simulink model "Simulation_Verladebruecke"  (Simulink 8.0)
settings: Solver=ode23  StartTime=0.0  StopTime=20  RelTol=1e-3
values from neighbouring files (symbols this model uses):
  cT = [1,0,0,0]    [demoVerladebrueckeRiccati.m]
  g = 9.81    [demoVerladebrueckeRiccati.m]
  k = R^(-1)*b'*P0    [demoVerladebrueckeRiccati.m]
  L = 10    [demoVerladebrueckeRiccati.m]
  M = -(cT*(A-b*k)^(-1)*b)^(-1)    [demoVerladebrueckeRiccati.m]
  mG = 1000    [demoVerladebrueckeRiccati.m]
  mK = 500    [demoVerladebrueckeRiccati.m]

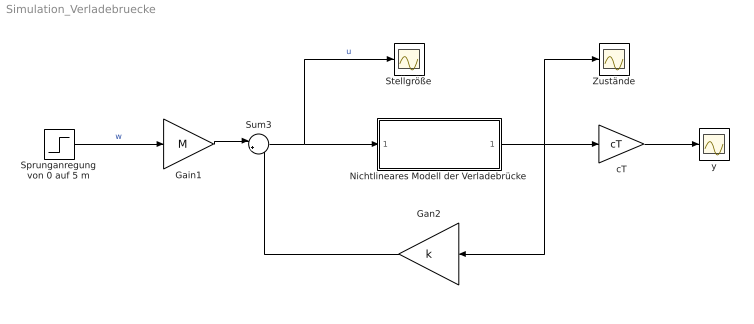
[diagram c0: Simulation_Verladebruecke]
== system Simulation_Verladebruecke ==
  Gain1 : Gain  Gain=M
  Gan2 : Gain  Gain=k  Multiplication=Matrix(K*u)
  Nichtlineares Modell der Verladebrücke : Subsystem
  Sprunganregung von 0 auf 5 m : Step  After=5  SampleTime=0
  Stellgröße : Scope
  Sum3 : Sum  Inputs=|+-
  Zustände : Scope
  cT : Gain  Gain=cT  Multiplication=Matrix(K*u)
  y : Scope
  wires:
  Sum3/1 -> Stellgröße/1, Nichtlineares Modell der Verladebrücke/1(Fk)  "u"
  Gan2/1 -> Sum3/2
  Gain1/1 -> Sum3/1
  Sprunganregung von 0 auf 5 m/1 -> Gain1/1  "w"
  cT/1 -> y/1
  Nichtlineares Modell der Verladebrücke/1(x) -> Zustände/1, cT/1, Gan2/1

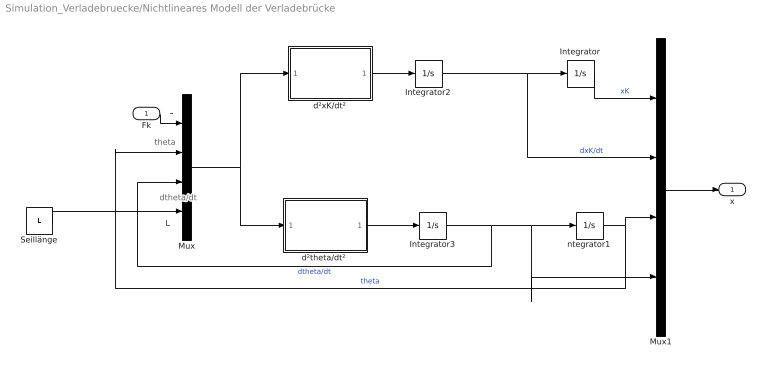
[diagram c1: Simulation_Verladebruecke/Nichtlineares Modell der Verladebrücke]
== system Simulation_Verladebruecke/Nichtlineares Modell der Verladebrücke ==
  note: L
  note: dtheta/dt
  note: theta
  Fk : Inport
  Integrator : Integrator
  Integrator2 : Integrator
  Integrator3 : Integrator  InitialCondition=0.0001
  Mux : Mux
  Mux1 : Mux
  Seillänge : Constant  Value=L
  "d²theta/dt² " : Subsystem
  d²xK/dt² : Subsystem
  ntegrator1 : Integrator
  x : Outport
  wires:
  Seillänge/1 -> Mux/4
  d²xK/dt²/1(Out1) -> Integrator2/1
  Integrator/1 -> Mux1/1  "xK"
  Mux1/1 -> x/1
  Integrator3/1 -> Mux1/4, ntegrator1/1, Mux/3  "dtheta/dt"
  Mux/1 -> d²xK/dt²/1(In1), "d²theta/dt² "/1(In1)
  "d²theta/dt² "/1(Out1) -> Integrator3/1
  Integrator2/1 -> Mux1/2, Integrator/1  "dxK/dt"
  ntegrator1/1 -> Mux1/3, Mux/2  "theta"
  Fk/1 -> Mux/1  "F"

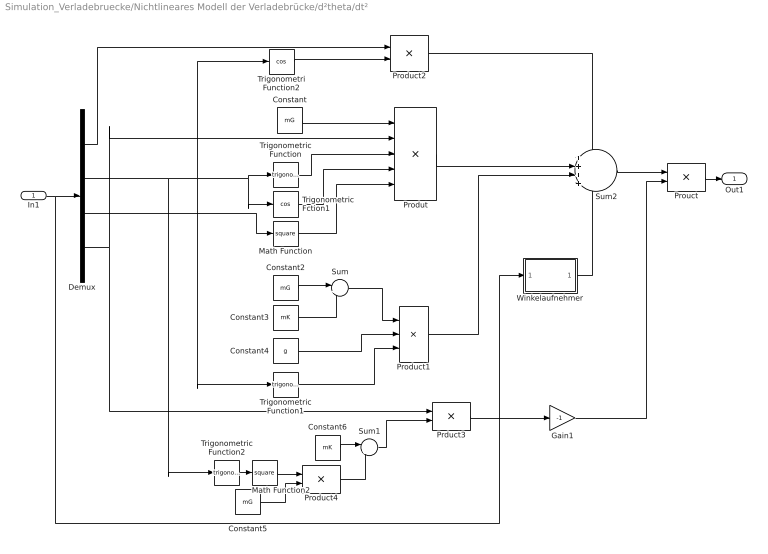
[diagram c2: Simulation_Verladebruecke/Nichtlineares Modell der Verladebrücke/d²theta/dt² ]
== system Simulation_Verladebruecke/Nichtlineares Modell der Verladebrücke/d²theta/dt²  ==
  In1 : Inport
  Constant : Constant  Value=mG
  Constant2 : Constant  Value=mG
  Constant3 : Constant  Value=mK
  Constant4 : Constant  Value=g
  Constant5 : Constant  Value=mG
  Constant6 : Constant  Value=mK
  Demux : Demux
  Gain1 : Gain  Gain=-1
  Math Function : Math  Operator=square
  Math Function2 : Math  Operator=square
  Prduct3 : Product
  Product1 : Product  Inputs=3
  Product2 : Product
  Product4 : Product
  Produt : Product  Inputs=5
  Prouct : Product  Inputs=*/
  Sum : Sum  Inputs=|++
  Sum1 : Sum  Inputs=|++
  Sum2 : Sum  Inputs=++++
  Trigonometri Function2 : Trigonometry  Operator=cos
  Trigonometric Fction1 : Trigonometry  Operator=cos
  Trigonometric Function : Trigonometry
  Trigonometric Function1 : Trigonometry
  Trigonometric Function2 : Trigonometry
  Winkelaufnehmer : Subsystem
  Out1 : Outport
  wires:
  Produt/1 -> Sum2/2
  Winkelaufnehmer/1(Out1) -> Sum2/4
  Demux/4 -> Produt/2, Prduct3/1
  In1/1 -> Winkelaufnehmer/1(In1), Demux/1
  Gain1/1 -> Prouct/2
  Prduct3/1 -> Gain1/1
  Prouct/1 -> Out1/1
  Sum2/1 -> Prouct/1
  Product1/1 -> Sum2/3
  Product2/1 -> Sum2/1
  Sum1/1 -> Prduct3/2
  Product4/1 -> Sum1/2
  Constant6/1 -> Sum1/1
  Constant5/1 -> Product4/2
  Math Function2/1 -> Product4/1
  Trigonometric Function2/1 -> Math Function2/1
  Trigonometri Function2/1 -> Product2/2
  Demux/1 -> Product2/1
  Trigonometric Function1/1 -> Product1/3
  Trigonometric Fction1/1 -> Produt/4
  Constant4/1 -> Product1/2
  Sum/1 -> Product1/1
  Constant3/1 -> Sum/2
  Constant2/1 -> Sum/1
  Demux/2 -> Trigonometric Function2/1, Trigonometri Function2/1, Trigonometric Function1/1, Trigonometric Fction1/1, Trigonometric Function/1
  Demux/3 -> Math Function/1
  Math Function/1 -> Produt/5
  Trigonometric Function/1 -> Produt/3
  Constant/1 -> Produt/1

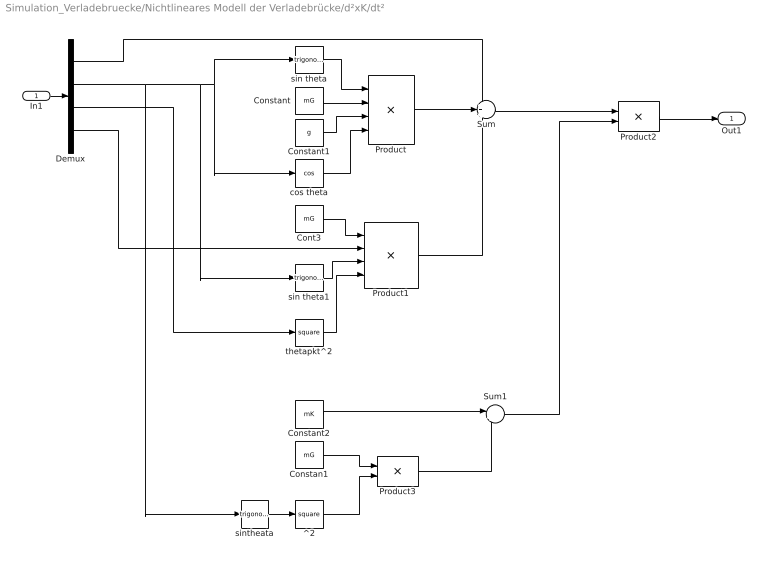
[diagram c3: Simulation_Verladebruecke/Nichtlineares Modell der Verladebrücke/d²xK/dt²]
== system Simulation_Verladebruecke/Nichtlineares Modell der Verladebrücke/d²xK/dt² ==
  In1 : Inport
  Constan1 : Constant  Value=mG
  Constant : Constant  Value=mG
  Constant1 : Constant  Value=g
  Constant2 : Constant  Value=mK
  Cont3 : Constant  Value=mG
  Demux : Demux
  Product : Product  Inputs=4
  Product1 : Product  Inputs=4
  Product2 : Product  Inputs=*/
  Product3 : Product
  Sum : Sum  Inputs=+++
  Sum1 : Sum  Inputs=|++
  ^2 : Math  Operator=square
  cos theta : Trigonometry  Operator=cos
  sin theta : Trigonometry
  sin theta1 : Trigonometry
  sintheata : Trigonometry
  thetapkt^2 : Math  Operator=square
  Out1 : Outport
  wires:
  Demux/4 -> Product1/2
  In1/1 -> Demux/1
  Sum1/1 -> Product2/2
  sin theta1/1 -> Product1/3
  Constant1/1 -> Product/3
  Constant2/1 -> Sum1/1
  Product3/1 -> Sum1/2
  ^2/1 -> Product3/2
  Constan1/1 -> Product3/1
  sintheata/1 -> ^2/1
  Product2/1 -> Out1/1
  Sum/1 -> Product2/1
  Demux/3 -> thetapkt^2/1
  Product1/1 -> Sum/3
  Product/1 -> Sum/2
  Demux/1 -> Sum/1
  thetapkt^2/1 -> Product1/4
  Cont3/1 -> Product1/1
  Constant/1 -> Product/2
  Demux/2 -> sintheata/1, sin theta1/1, cos theta/1, sin theta/1
  cos theta/1 -> Product/4
  sin theta/1 -> Product/1

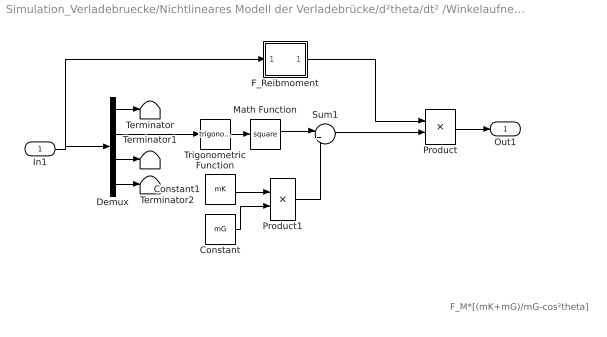
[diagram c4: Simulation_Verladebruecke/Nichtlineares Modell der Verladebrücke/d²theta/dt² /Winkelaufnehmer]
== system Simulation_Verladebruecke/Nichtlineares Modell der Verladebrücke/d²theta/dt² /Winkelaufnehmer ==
  note: F_M*[(mK+mG)/mG-cos²theta]
  In1 : Inport
  Constant : Constant  Value=mG
  Constant1 : Constant  Value=mK
  Demux : Demux
  F_Reibmoment : Subsystem
  Math Function : Math  Operator=square
  Product : Product
  Product1 : Product  Inputs=*/
  Sum1 : Sum  Inputs=|++
  Terminator : Terminator
  Terminator1 : Terminator
  Terminator2 : Terminator
  Trigonometric Function : Trigonometry
  Out1 : Outport
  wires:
  Product1/1 -> Sum1/2
  Demux/4 -> Terminator2/1
  Product/1 -> Out1/1
  F_Reibmoment/1(Out1) -> Product/1
  Sum1/1 -> Product/2
  Math Function/1 -> Sum1/1
  Constant/1 -> Product1/2
  Constant1/1 -> Product1/1
  Trigonometric Function/1 -> Math Function/1
  Demux/2 -> Trigonometric Function/1
  Demux/3 -> Terminator1/1
  Demux/1 -> Terminator/1
  In1/1 -> F_Reibmoment/1(In1), Demux/1

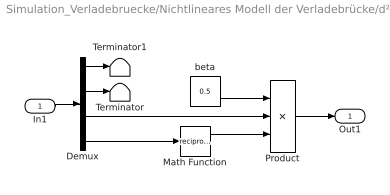
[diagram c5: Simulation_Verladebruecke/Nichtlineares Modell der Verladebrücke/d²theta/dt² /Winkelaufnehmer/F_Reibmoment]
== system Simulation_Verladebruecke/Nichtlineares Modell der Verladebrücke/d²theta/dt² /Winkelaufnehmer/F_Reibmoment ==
  In1 : Inport
  Demux : Demux
  Math Function : Math  Operator=reciprocal
  Product : Product  Inputs=3
  Terminator : Terminator
  Terminator1 : Terminator
  beta : Constant  Value=0.5
  Out1 : Outport
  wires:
  Demux/1 -> Terminator1/1
  Math Function/1 -> Product/3
  beta/1 -> Product/1
  Demux/4 -> Math Function/1
  Product/1 -> Out1/1
  Demux/2 -> Terminator/1
  Demux/3 -> Product/2
  In1/1 -> Demux/1
